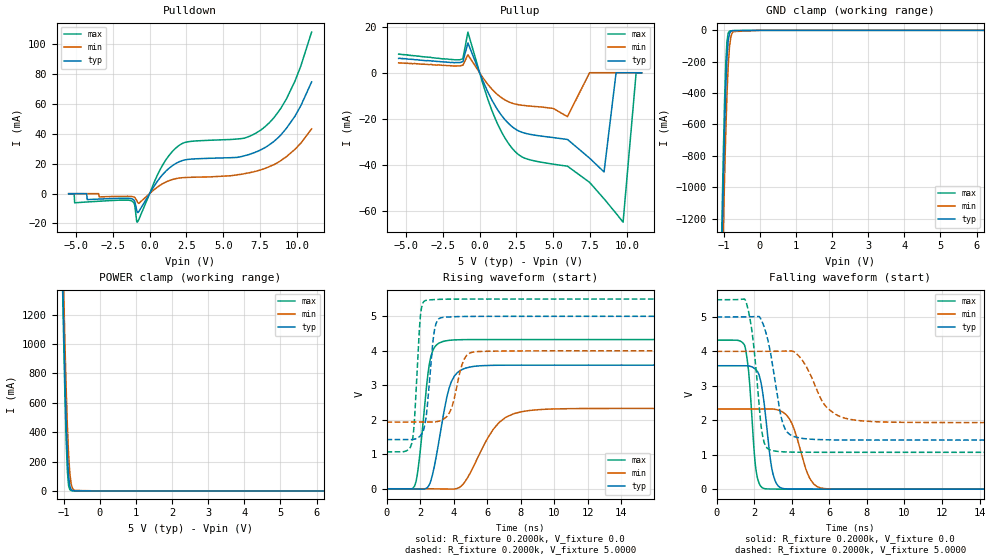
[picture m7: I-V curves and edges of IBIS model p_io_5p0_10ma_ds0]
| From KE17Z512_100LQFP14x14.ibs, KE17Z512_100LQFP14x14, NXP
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[Model] p_io_5p0_10ma_ds0
|   Model p_io_5p0_10ma_ds0
| This model was characterised for following simulation conditions:
| External (pad) voltage:
|   - Typ: 5.0V,   - Min: 4.0V,   - Max: 5.5V
| Library cells for typ/min/max conditions are connected as defined below:
|  pad - External Pad
|  ipp_do_lv - Core Input
|  ipp_obe_lv - Output Buffer Enable
|  abt_close_nor_rst_mv - vdde
|  dvdd - dvdd
|  dvss - dvss
|  esd_boost - vdde
|  ipp_dse_lv - dvss
|  ipp_ina_280_mv - NC
|  ipp_ina_40_a_mv - NC
|  ipp_ina_40_b_mv - NC
|  ipp_ina_40_c_mv - NC
|  ipp_ina_40_d_mv - NC
|  ipp_ina_40_e_mv - NC
|  ipp_ina_40_f_mv - NC
|  ipp_ina_40_g_mv - NC
|  ipp_ina_40_h_mv - NC
|  ipp_ind_lv - NC
|  ipp_sre_lv - dvss
|  vdde - vdde
|  vsse - vsse
| All other pins connected to ground
Model_type I/O
Polarity   Non-Inverting
Enable   Active-High
Vinl =   1.5000V
Vinh =   3.5000V
Vmeas =  2.5000V
Cref =   50.0000F
C_comp   1.9155pF   1.8351pF   2.0353pF
[Model Spec]
| variable   typ   min   max
Vinh   3.5000V   2.8000V   3.8500V
Vinl   1.5000V   1.2000V   1.6500V
S_overshoot_high   5.3000V   4.3000V   5.8000V
S_overshoot_low   -0.3000V   -0.3000V   -0.3000V
Vmeas   2.5000V   2.0000V   2.7500V
[Temperature Range]   25.0000   0.1250k   -40.0000
[Voltage Range]   5.0000V   4.0000V   5.5000V
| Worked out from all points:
|   slope of the pulldown table from 0 to 0.75 V, typ, clamps not added: 66.9 ohm
|   slope of the pullup table from 0 to 0.75 V, typ, clamps not added: 69.2 ohm
|   POWER clamp passes 1 mA (typ) near -0.72 V on its own axis
|   rising waveform, R_fixture 0.2000k, V_fixture 0.0: 20-80 % time 825ps typ, 1.61ns min, 549ps max; typ from 0 V to 3.58 V
|   rising waveform, R_fixture 0.2000k, V_fixture 5.0000: 20-80 % time 395ps typ, 615ps min, 300ps max; typ from 1.43 V to 5 V
|   falling waveform, R_fixture 0.2000k, V_fixture 0.0: 20-80 % time 468ps typ, 792ps min, 338ps max; typ from 3.58 V to 0 V
|   falling waveform, R_fixture 0.2000k, V_fixture 5.0000: 20-80 % time 670ps typ, 1.17ns min, 467ps max; typ from 5 V to 1.43 V
[Pulldown]
|Voltage   I(typ)   I(min)   I(max)
-5.5V     -10uA      10uA       -150uA
-5.126V   -10uA      10uA       -210uA
-5.092V   -20uA      0A         -6.13mA
-1.216V   -3.461mA   -1.919mA   -4.884mA
-1.012V   -5.066mA   -2.53mA    -7.744mA
-842mV    -12.47mA   -5.416mA   -19.14mA
722mV     10.88mA    5.707mA    16.32mA
1.912V    20.93mA    10.3mA     31.67mA
6.434V    25.37mA    13.4mA     37.19mA
8.304V    34mA       18.9mA     49.4mA
9.868V    51.9mA     29.7mA     75.4mA
11V       74.9mA     43.4mA     108.3mA
[Pullup]
|Voltage   I(typ)   I(min)   I(max)
-5.5V     6.2mA      4.3mA      8.1mA
-1.342V   4.4mA      2.98mA     5.63mA
-798mV    12.97mA    7.775mA    17.65mA
834mV     -11.9mA    -7.156mA   -16.44mA
2.16V     -23.2mA    -13.14mA   -32.45mA
5.968V    -29mA      -19.1mA    -40.62mA
7.464V    -37.1mA    0A         -47.61mA
8.45V     -43.12mA   10uA       -54.79mA
9.266V    -40uA      10uA       -61.1mA
9.742V    -20uA      0A         -64.94mA
10.63V    -10uA      0A         -220uA
11V       -20uA      -10uA      -160uA
[GND_clamp]
|Voltage   I(typ)   I(min)   I(max)
-5.5V     -66.54A    -66.41A    -66.68A
-1.08V    -1.754A    -2.051A    -1.581A
-1.046V   -1.352A    -1.659A    -1.169A
-1.012V   -977.4mA   -1.289A    -787.6mA
-978mV    -643.1mA   -949.6mA   -456.8mA
-944mV    -367.9mA   -651.2mA   -207.4mA
-910mV    -172.9mA   -405.7mA   -67.09mA
-876mV    -65.09mA   -224mA     -17.43mA
-842mV    -21.2mA    -108.6mA   -5.66mA
-740mV    -1.706mA   -8.008mA   -2.163mA
0V        -49.35pA   -428.8pA   -500.7pA
11V       0A         0A         0A
[POWER_clamp]
|Voltage   I(typ)   I(min)   I(max)
-5.5V     67.36A     67.1A      67.58A
-1.036V   1.535A     1.738A     1.426A
-1.002V   1.145A     1.361A     1.021A
-968mV    787.9mA    1.014A     654.2mA
-934mV    481mA      703.8mA    347.7mA
-900mV    245.7mA    444.9mA    136.4mA
-866mV    99.48mA    249.2mA    36.93mA
-832mV    32.56mA    121.8mA    8.258mA
-798mV    9.635mA    52.79mA    2.194mA
-696mV    574.4uA    3.321mA    568.6uA
0V        105.1pA    1.642nA    92.78pA
11V       0A         0A         0A
[Ramp]
| variable   typ   min   max
dV/dt_r  2.1507/0.8251n   1.3974/1.6080n   2.5959/0.5485n
dV/dt_f  2.1449/0.6698n   1.2405/1.1739n   2.6581/0.4674n
R_load = 0.2000k
[Rising Waveform]
R_fixture= 0.2000k
V_fixture= 0.0
V_fixture_min= 0.0
V_fixture_max= 0.0
|time   V(typ)   V(min)   V(max)
0s        2.085nV    24.17nV    15.65nV
1.676ns   -3.823mV   74.01uV    83.96mV
1.937ns   -7.582mV   107.3uV    779.7mV
2.637ns   222.9mV    -846.6uV   3.821V
3.484ns   2.389V     -7.504mV   4.285V
3.866ns   3.106V     -11.89mV   4.31V
4.518ns   3.46V      106.8mV    4.323V
6.712ns   3.581V     1.923V     4.326V
8.339ns   3.584V     2.257V     4.327V
40ns      3.584V     2.329V     4.327V
[Rising Waveform]
R_fixture= 0.2000k
V_fixture= 5.0000
V_fixture_min= 4.0000
V_fixture_max= 5.5000
|time   V(typ)   V(min)   V(max)
0s        1.425V     1.933V     1.07V
1.497ns   1.425V     1.932V     1.303V
1.661ns   1.437V     1.932V     1.966V
2.024ns   1.539V     1.931V     5.024V
2.341ns   2.021V     1.93V      5.461V
2.874ns   4.64V      1.938V     5.486V
3.354ns   4.969V     2.004V     5.495V
4.625ns   4.995V     3.753V     5.5V
5.271ns   4.998V     3.972V     5.5V
40ns      5V         4V         5.5V
[Falling Waveform]
R_fixture= 0.2000k
V_fixture= 0.0
V_fixture_min= 0.0
V_fixture_max= 0.0
|time   V(typ)   V(min)   V(max)
0s        3.584V     2.329V     4.327V
1.496ns   3.586V     2.329V     4.171V
1.709ns   3.579V     2.329V     3.413V
2.117ns   3.456V     2.329V     493.5mV
2.523ns   2.541V     2.33V      18.05mV
3.002ns   446.9mV    2.326V     3.337mV
3.614ns   12.45mV    2.203V     1.117mV
4.983ns   1.142mV    293mV      181uV
5.702ns   459.7uV    19.18mV    88.31uV
40ns      2.13uV     5.857uV    96.62nV
[Falling Waveform]
R_fixture= 0.2000k
V_fixture= 5.0000
V_fixture_min= 4.0000
V_fixture_max= 5.5000
|time   V(typ)   V(min)   V(max)
0s        5V         4V         5.5V
1.552ns   5.001V     4V         5.461V
1.899ns   5.008V     4V         4.54V
2.463ns   4.813V     4V         1.51V
3.059ns   3.321V     4.002V     1.11V
3.657ns   1.739V     4.011V     1.081V
4.92ns    1.454V     3.408V     1.071V
5.859ns   1.433V     2.379V     1.07V
7.719ns   1.426V     1.984V     1.07V
40ns      1.425V     1.933V     1.07V
